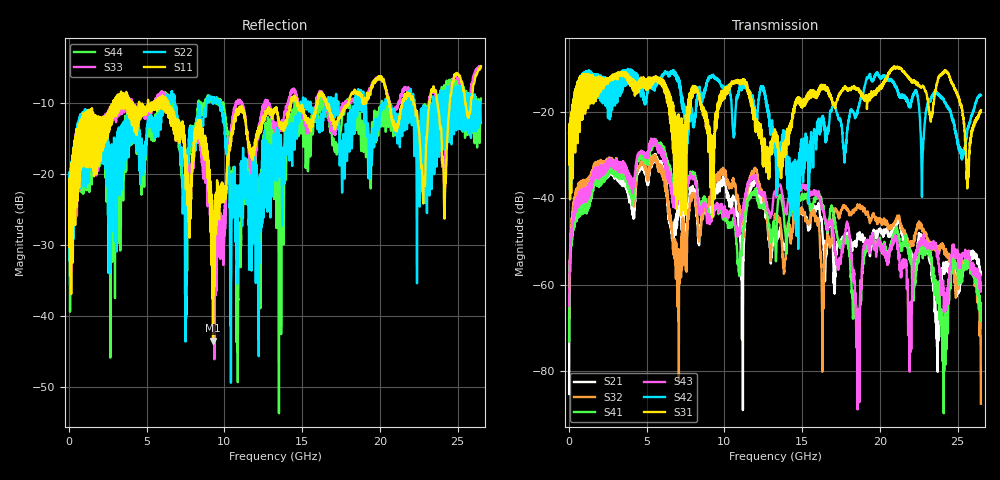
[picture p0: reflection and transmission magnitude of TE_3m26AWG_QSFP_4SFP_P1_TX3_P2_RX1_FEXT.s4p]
!Agilent Technologies,N5222A,MY51421691,A.10.00.00
!Agilent N5222A: A.10.00.00
!Date: Friday, January 30, 2015 12:37:28
!Correction: S11(Full 4 Port(1,2,3,4))
!S12(Full 4 Port(1,2,3,4))
!S13(Full 4 Port(1,2,3,4))
!S14(Full 4 Port(1,2,3,4))
!S21(Full 4 Port(1,2,3,4))
!S22(Full 4 Port(1,2,3,4))
!S23(Full 4 Port(1,2,3,4))
!S24(Full 4 Port(1,2,3,4))
!S31(Full 4 Port(1,2,3,4))
!S32(Full 4 Port(1,2,3,4))
!S33(Full 4 Port(1,2,3,4))
!S34(Full 4 Port(1,2,3,4))
!S41(Full 4 Port(1,2,3,4))
!S42(Full 4 Port(1,2,3,4))
!S43(Full 4 Port(1,2,3,4))
!S44(Full 4 Port(1,2,3,4))
!S4P File: Measurements: <S11,S12,S13,S14>,
!<S21,S22,S23,S24>,
!<S31,S32,S33,S34>,
!<S41,S42,S43,S44>:
# Hz S  dB  R 50.0
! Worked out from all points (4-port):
!   2650 points, 10 MHz to 26.5 GHz, reference 50 ohm
!   strongest paths, dB at 10 MHz, 6.63 GHz, 13.26 GHz, 19.88 GHz, 26.5 GHz:
!     S31: -25.0, -17.7, -24.8, -15.2, -19.6
!     S42: -24.8, -11.2, -27.4, -11.2, -16.2
!     S43: -65.0, -39.7, -38.5, -49.7, -60.4
!     S41: -73.2, -37.2, -48.6, -49.6, -64.3
!     S32: -67.9, -48.6, -44.2, -45.1, -87.6
!     S21: -85.4, -49.4, -47.3, -48.2, -57.5
!   lowest |S11| = -43.4 dB at 9.27 GHz (marker M1), VSWR 1.01, Z = 50.1 + j0.672 ohm
!   |S11| at or under -10 dB: start of sweep to 2.858 GHz; 6.4 GHz to 14.25 GHz (7.851 GHz wide, 76 % of centre); 16.59 GHz to 18.01 GHz (1.418 GHz wide, 8.2 % of centre)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
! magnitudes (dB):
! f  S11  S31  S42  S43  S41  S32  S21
! 10 MHz  -20.8  -25.0  -24.8  -65.0  -73.2  -67.9  -85.4
! 1.74 GHz  -11.8  -12.0  -11.3  -35.2  -36.9  -34.2  -36.4
! 9.27 GHz  -43.4  -27.7  -11.6  -43.2  -43.3  -38.0  -40.5
! 10.9 GHz  -10.9  -13.3  -16.2  -47.2  -55.2  -41.3  -46.1
! 14.32 GHz  -9.7  -22.0  -42.7  -39.9  -42.9  -48.8  -47.9
! 18.58 GHz  -8.8  -14.9  -19.7  -76.2  -72.6  -41.8  -48.5
! 26.5 GHz  -4.8  -19.6  -16.2  -60.4  -64.3  -87.6  -57.5
